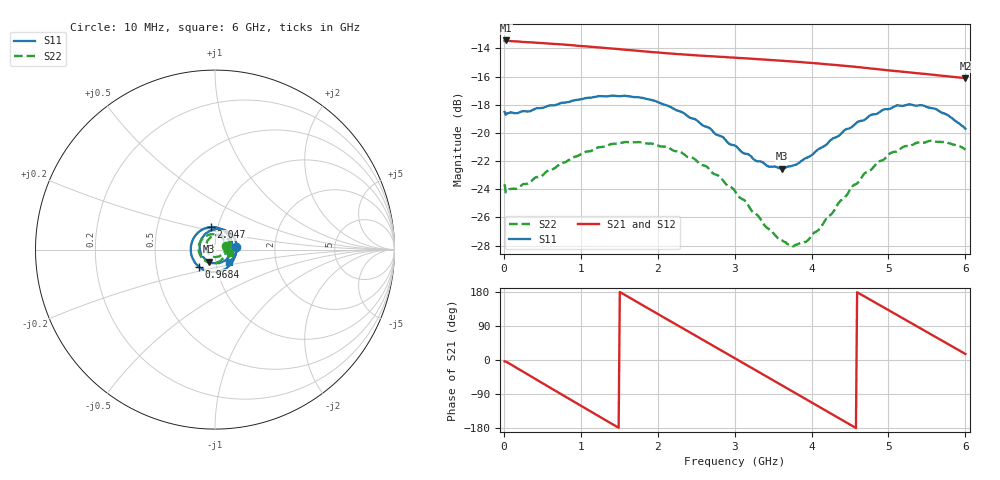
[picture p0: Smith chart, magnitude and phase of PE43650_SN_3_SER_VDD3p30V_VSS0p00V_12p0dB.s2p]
!Keysight Technologies,N5245B,MY57181451,A.13.50.07
!Date: Tuesday, May 07, 2019 08:00:09
!Correction: S11(Full 2 Port(1,2))
!S21(Full 2 Port(1,2))
!S12(Full 2 Port(1,2))
!S22(Full 2 Port(1,2))
!S2P File: Measurements: S11, S21, S12, S22:
# Hz S  dB  R 50
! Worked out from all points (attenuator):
!   401 points, 10 MHz to 6 GHz, reference 50 ohm
!   highest |S21| = -13.44 dB at 24.98 MHz (marker M1); lowest = -16.1 dB at 6 GHz (marker M2)
!   lowest |S11| = -22.5 dB at 3.619 GHz (marker M3), VSWR 1.16, Z = 46.5 - j6.29 ohm
!   |S11| at or under -10 dB: start of sweep to end of sweep
!   |S22| runs from -28.0 to -20.6 dB; largest |S21 - S12| = 0.0017
!   S11 on the Smith chart (normalised r, x): 10 MHz: 1.27, +0.03; 968.4 MHz: 0.82, -0.16; 2.047 GHz: 0.93, +0.24; 6 GHz: 1.16, -0.16
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1e7  -18.52 6.2  -13.46 -3.5  -13.47 -3.2  -23.65 16.4
2.4975e7  -18.72 -0.3  -13.44 -4.3  -13.50 -4.1  -24.23 4.3
2.64575e8  -18.46 -38.7  -13.55 -32.6  -13.59 -32.6  -23.63 -38.9
5.34125e8  -18.17 -76.7  -13.64 -65.0  -13.69 -65.0  -22.86 -77.6
9.684e8  -17.65 -133.2  -13.82 -116.8  -13.87 -116.8  -21.62 -131.4
1.013325e9  -17.61 -138.9  -13.84 -122.1  -13.89 -122.1  -21.48 -136.7
1.2679e9  -17.39 -169.6  -13.95 -152.3  -14.01 -152.3  -21.01 -164.7
1.5075e9  -17.39 161.9  -14.06 179.5  -14.12 179.4  -20.73 169.5
1.7471e9  -17.48 134.3  -14.18 151.3  -14.24 151.3  -20.65 145.0
2.01665e9  -17.84 103.7  -14.30 119.8  -14.36 119.8  -20.92 117.8
2.0466e9  -17.92 100.1  -14.32 116.2  -14.37 116.3  -20.97 114.5
2.480875e9  -19.02 48.8  -14.49 65.6  -14.54 65.7  -21.86 70.4
2.750425e9  -20.09 15.5  -14.58 34.2  -14.64 34.2  -22.96 40.9
3.005e9  -20.90 -19.3  -14.67 4.4  -14.72 4.5  -24.14 11.6
3.289525e9  -22.01 -62.0  -14.77 -28.8  -14.82 -28.7  -25.81 -27.3
3.618975e9  -22.53 -115.6  -14.89 -67.3  -14.93 -67.3  -27.65 -80.7
3.768725e9  -22.31 -140.4  -14.94 -84.9  -14.99 -84.8  -28.05 -108.3
4.008325e9  -21.56 -177.9  -15.04 -112.9  -15.09 -112.9  -27.25 -152.5
4.517475e9  -19.60 113.6  -15.29 -172.5  -15.34 -172.3  -23.88 132.5
5.01165e9  -18.30 57.6  -15.57 130.1  -15.62 130.3  -21.50 78.0
5.475875e9  -18.10 10.1  -15.82 76.4  -15.87 76.5  -20.69 33.6
6e9  -19.70 -40.6  -16.12 15.9  -16.16 16.0  -21.19 -11.7
